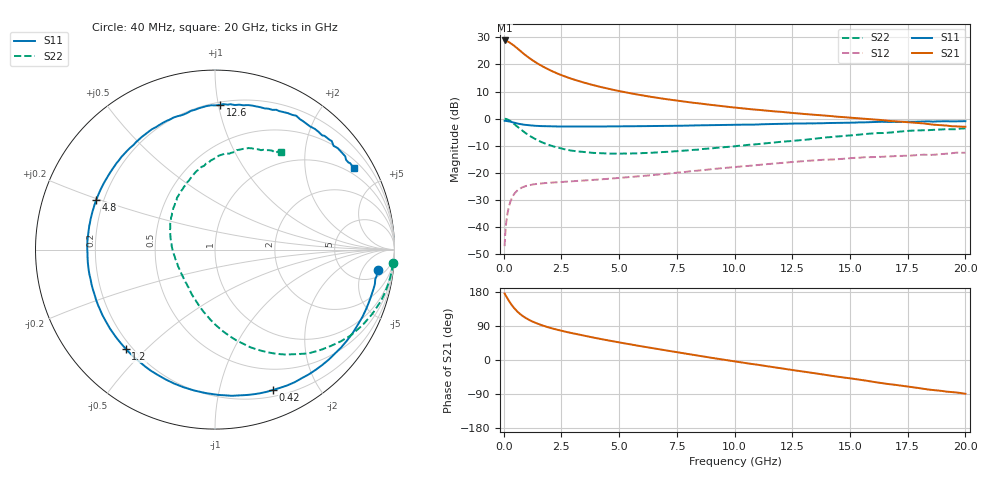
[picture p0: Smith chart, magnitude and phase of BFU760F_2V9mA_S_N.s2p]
! Filename:  P:\Prog\Test\Noise\ATS_data\Testdata_Net\BFU760\BFU760F_2W_C1_2V9mA_D.s2p
! Date/Time: Mon 06/Feb/2012 15:05:15
! BFU760_2W_C1_2V_9mA
! bias mode 1: Vout= 2.0002 V, Iout= 9.0250 mA, Vin= 0.7705 V, Iin= 0.0259 mA
! Date/time Fri Mar 18 11:26:21 2011
! Device data file deembeded for feedlines and parallel
! Original file: \BFU760\BFU760_2W_C1_2V9mA_R.s2p
! Feed-files: PR003V01_101208_Feed1.s2p, PR003V01_101208_Feed2.s2p
! Parallel-file: PR003V01_101208_Par.s2p
# MHz S MA R 50
!  Freq-MHz  S11-mag  S11-arg  S21-mag  S21-arg  S12-mag  S12-arg  S22-mag  S22-arg
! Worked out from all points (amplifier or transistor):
!   167 points, 40 MHz to 20 GHz, reference 50 ohm
!   highest |S21| = 28.9 dB at 40 MHz (marker M1)
!   |S21| within 3 dB of that: start of sweep to 600.4 MHz
!   unconditionally stable (mu >= 1): 5.376 GHz to 13.17 GHz; 13.28 GHz to 13.45 GHz
!   at 550 MHz: K = 0.12, MSG = 26.6 dB, |S12| = -26.9 dB
!   at 4.2 GHz: K = 0.86, MSG = 17.1 dB, |S12| = -22.5 dB
!   at 20 GHz: K = 0.83, MSG = 4.8 dB, |S12| = -12.6 dB
!   lowest NFmin = 0.44 dB at 850 MHz
!   S11 on the Smith chart (normalised r, x): 40 MHz: 8, -10; 420 MHz: 0.27, -1.46; 1.2 GHz: 0.18, -0.43; 4.8 GHz: 0.17, +0.20; 12.6 GHz: 0.22, +1.01; 20 GHz: 0.77, +3.52
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40  0.9126 -7.1  27.77 175.7  0.004383 84.9  0.994 -4.5
50  0.9125 -9.3  27.76 174.0  0.005551 79.5  0.9928 -5.7
60  0.9079 -10.4  27.4 173.2  0.006374 83.2  0.9923 -6.7
140  0.9031 -24.4  27.01 164.8  0.0151 77.2  0.972 -15.8
240  0.8844 -41.1  25.78 154.7  0.02478 68.8  0.9265 -26.4
340  0.8641 -56.1  24 145.8  0.03289 61.2  0.8669 -36.2
420  0.8458 -67.6  22.78 139.4  0.03831 56.0  0.8161 -42.9
600  0.8095 -88.9  19.67 127.4  0.04711 46.3  0.7039 -56.1
800  0.7801 -107.1  16.65 117.2  0.05335 38.7  0.6014 -67.5
1000  0.7585 -121.0  14.22 109.3  0.05722 33.4  0.5209 -76.6
1200  0.7435 -132.0  12.35 102.9  0.05986 29.7  0.4592 -84.2
1550  0.7281 -146.4  9.931 94.0  0.06284 25.3  0.3826 -95.0
1950  0.7172 -158.4  8.056 85.9  0.06503 22.3  0.3268 -105.4
2500  0.713 -170.6  6.349 77.2  0.06741 20.3  0.2798 -117.8
3400  0.712 174.8  4.726 65.2  0.07132 18.8  0.243 -133.7
4800  0.7176 157.2  3.359 48.7  0.07868 18.3  0.2259 -155.9
6800  0.7309 137.0  2.368 27.6  0.09329 16.9  0.2387 177.9
10200  0.7711 107.5  1.568 -5.5  0.1291 7.7  0.315 139.4
12600  0.8066 88.0  1.259 -27.3  0.1585 -3.5  0.3898 116.4
13400  0.8129 82.2  1.18 -34.2  0.1682 -8.6  0.4207 108.9
16800  0.8675 55.5  0.8988 -64.3  0.2004 -29.2  0.554 78.7
20000  0.8957 30.4  0.7055 -89.1  0.2335 -51.2  0.6589 55.9
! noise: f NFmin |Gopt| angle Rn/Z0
400  0.4483  0.2117  17.97  0.0659
700  0.4441  0.2038  45.61  0.0648
1100  0.444  0.2317  74.47  0.0624
1500  0.4504  0.2711  94.15  0.0592
1900  0.4631  0.3075  109.1  0.0555
2350  0.4851  0.3428  123.5  0.0509
3000  0.5311  0.389  142.4  0.0443
3800  0.6108  0.4501  163.1  0.0375
4600  0.716  0.5147  180  0.034
6000  0.9616  0.5684  200.7  0.0413
